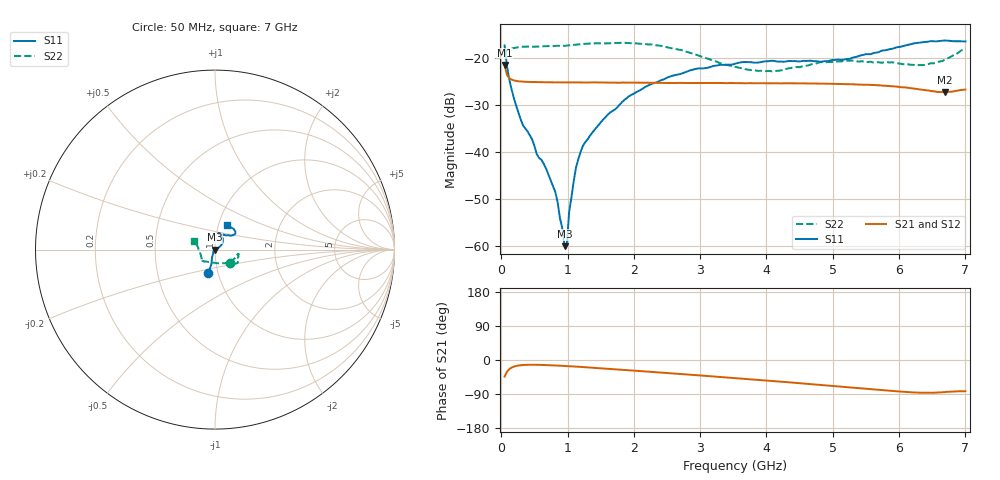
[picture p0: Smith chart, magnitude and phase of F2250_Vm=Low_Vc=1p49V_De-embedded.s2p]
! Integrated Device Technology
! Corporate Headquarters
! 6024 Silver Creek Valley Road
! San Jose, CA 95138  USA
! Phone:  1-408-284-8200
! Toll Free:  1-800-223-1366
! Webpage:  http://www.idt.com/
! Timing and RF Division
! 515 Groton Road, Suite 102
! Westford, MA 01886-6024
! Device:  F2250
! Description: Voltage Variable RF Attenuator
! Frequency:  50.0 -  6000.00 MHz
! Package:  3x3 mm Thin QFN Plastic Package: 16 pin
! Ports:  2 RF, 3 DC
!  Pin  1  = GND
!  Pin  2  = NC
!  Pin  3  = RF1  = Port 1
!  Pin  4  = NC
!  Pin  5  = GND
!  Pin  6  = GND
!  Pin  7  = GND
!  Pin  8  = GND
!  Pin  9  = NC
!  Pin 10  = RF2  = Port 2
!  Pin 11  = NC
!  Pin 12  = GND
!  Pin 13  = GND
!  Pin 14  = VCNTRL
!  Pin 15  = VDD
!  Pin 16  = VMODE
! Vcntrl:  1.490 Volts
! Vmode:  +0.000 Volts
! Vdd:  +3.30  Volts
! Current:  1.191 mA
! Data:  The device was measured on a the F2250 evaluation board which has
!  individual transmission lines to the RF pins.  Data was collected
!  using a calibrated network analyzer.  The evaluation board was
!  de-embedded using a TRL calibration technique.
!  The reference plane is the edge of the package pin.
! Misc:  SN 10
!  Action Tracker AT0258
! Date Measured:  2014-11-26
! Date:  2015-10-15  MJV
! Note:
!  Integrated Device Technology supplies this data as a sample of measured
!  data at the package pin for this product.  Your particular data for this
!  product may vary.
!  Data was taken at 25 degrees C.
!  Integrated Device Technology reserves the right to change this data at anytime.
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# GHz S dB R 50
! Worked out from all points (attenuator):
!   201 points, 50 MHz to 7 GHz, reference 50 ohm
!   highest |S21| = -21.39 dB at 50 MHz (marker M1); lowest = -27.2 dB at 6.687 GHz (marker M2)
!   lowest |S11| = -60.0 dB at 953.5 MHz (marker M3), VSWR 1.00, Z = 49.9 - j0.0591 ohm
!   |S11| at or under -10 dB: start of sweep to end of sweep
!   |S22| runs from -22.8 to -16.7 dB; largest |S21 - S12| = 0.00029
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0.05  -17.25 -106.1  -21.39 -43.7  -21.42 -43.8  -19.21 -41.1
0.1195  -24.41 -106.9  -24.22 -24.2  -24.21 -24.2  -18.00 -14.5
0.29325  -33.05 -116.1  -24.90 -13.8  -24.91 -13.8  -17.52 -10.9
0.6755  -43.49 -141.3  -25.09 -13.4  -25.08 -13.4  -17.40 -14.9
0.8145  -48.47 -175.1  -25.11 -14.5  -25.12 -14.5  -17.33 -17.6
0.91875  -56.12 144.5  -25.13 -15.4  -25.13 -15.4  -17.27 -19.8
0.9535  -60.04 -143.5  -25.12 -15.7  -25.13 -15.7  -17.34 -20.2
0.98825  -59.70 -15.9  -25.12 -16.0  -25.14 -16.0  -17.26 -20.6
1.023  -52.80 1.4  -25.13 -16.3  -25.13 -16.3  -17.21 -20.7
1.12725  -43.26 17.4  -25.12 -17.4  -25.13 -17.4  -17.06 -22.5
1.2315  -38.64 20.3  -25.12 -18.6  -25.12 -18.6  -16.92 -24.4
1.5095  -33.47 27.3  -25.13 -22.0  -25.14 -22.0  -16.81 -27.0
1.857  -28.86 32.8  -25.16 -26.2  -25.18 -26.2  -16.68 -30.5
2.37825  -24.85 42.4  -25.21 -32.8  -25.23 -32.7  -17.25 -35.0
2.93425  -22.24 56.6  -25.26 -39.9  -25.26 -39.9  -19.19 -44.2
3.525  -21.14 70.2  -25.27 -47.7  -25.27 -47.8  -21.80 -71.1
4.11575  -20.54 78.3  -25.31 -55.7  -25.29 -55.8  -22.74 -107.3
4.7065  -20.58 71.2  -25.33 -64.2  -25.33 -64.2  -21.21 -130.0
5.85325  -18.05 39.2  -25.89 -81.1  -25.91 -81.1  -20.88 -144.7
6.3745  -16.52 40.5  -26.72 -86.6  -26.70 -86.6  -21.42 -166.3
6.68725  -16.18 48.1  -27.22 -84.6  -27.23 -84.6  -20.26 170.7
7  -16.37 62.7  -26.64 -82.3  -26.61 -82.4  -17.88 158.5
